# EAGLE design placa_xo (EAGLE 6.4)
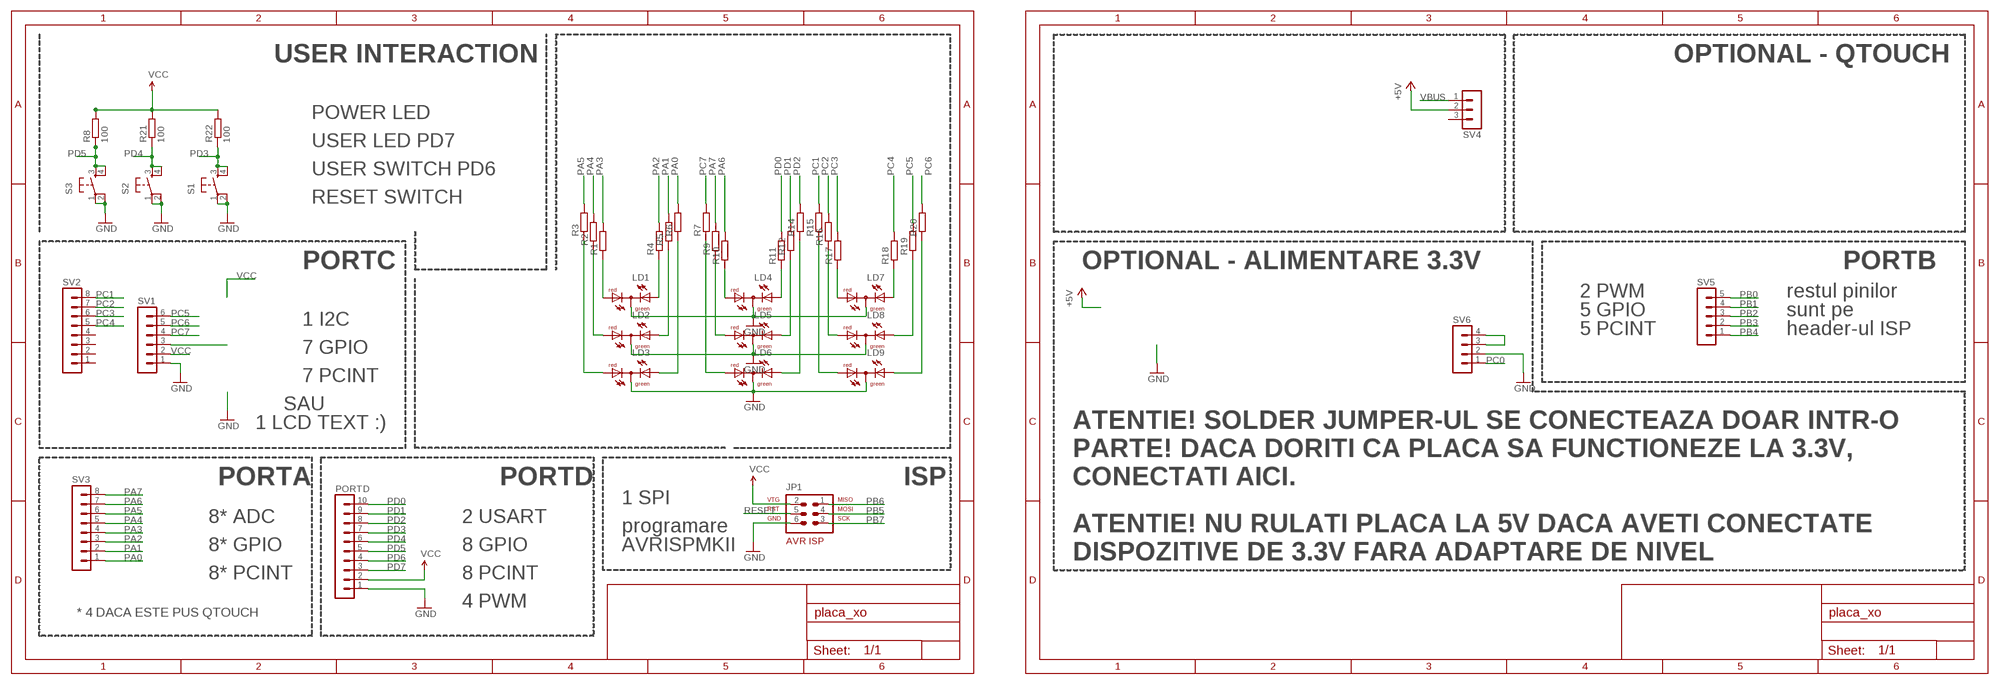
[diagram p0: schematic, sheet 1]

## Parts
JP1  AVR-ISP-6  [AVR-ISP-6]
LD1  DUOLED-RG-C  [DUOLED-C-5MM]
LD2  DUOLED-RG-C  [DUOLED-C-5MM]
LD3  DUOLED-RG-C  [DUOLED-C-5MM]
LD4  DUOLED-RG-C  [DUOLED-C-5MM]
LD5  DUOLED-RG-C  [DUOLED-C-5MM]
LD6  DUOLED-RG-C  [DUOLED-C-5MM]
LD7  DUOLED-RG-C  [DUOLED-C-5MM]
LD8  DUOLED-RG-C  [DUOLED-C-5MM]
LD9  DUOLED-RG-C  [DUOLED-C-5MM]
PORTD  MA10-1W  [MA10-1W]
R1  R-EU_M0805  [M0805]
R2  R-EU_M0805  [M0805]
R3  R-EU_M0805  [M0805]
R4  R-EU_M0805  [M0805]
R5  R-EU_M0805  [M0805]
R6  R-EU_M0805  [M0805]
R7  R-EU_M0805  [M0805]
R8  100  R-EU_0204/7  [0204/7]
R9  R-EU_M0805  [M0805]
R10  R-EU_M0805  [M0805]
R11  R-EU_M0805  [M0805]
R12  R-EU_M0805  [M0805]
R14  R-EU_M0805  [M0805]
R15  R-EU_M0805  [M0805]
R16  R-EU_M0805  [M0805]
R17  R-EU_M0805  [M0805]
R18  R-EU_M0805  [M0805]
R19  R-EU_M0805  [M0805]
R20  R-EU_M0805  [M0805]
R21  100  R-EU_0204/7  [0204/7]
R22  100  R-EU_0204/7  [0204/7]
S1  TAC_SWITCHPTH  [TACTILE-PTH]
S2  TAC_SWITCHPTH  [TACTILE-PTH]
S3  TAC_SWITCHPTH  [TACTILE-PTH]
SV1  MA06-1  [MA06-1]
SV2  MA08-1  [MA08-1]
SV3  MA08-1  [MA08-1]
SV4  MA03-1  [MA03-1]
SV5  MA05-1  [MA05-1]
SV6  MA04-1  [MA04-1]

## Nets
+5V: SV4.2
GND: JP1.6 LD1.C LD2.C LD3.C LD4.C LD5.C LD6.C LD7.C LD8.C LD9.C PORTD.1 S1.1 S1.2 S2.1 S2.2 S3.1 S3.2 SV1.1 SV6.2
N$5: SV6.3 SV6.4
N$7: LD1.AR R1.1
N$8: LD1.AX(AG) R4.1
N$9: LD2.AR R2.1
N$10: LD2.AX(AG) R5.1
N$11: LD3.AR R3.1
N$12: SV1.3
N$13: LD3.AX(AG) R6.1
N$14: LD6.AR R7.1
N$15: LD6.AX(AG) R14.1
N$16: LD5.AX(AG) R12.1
N$18: LD4.AX(AG) R11.1
N$19: LD4.AR R10.1
N$20: LD5.AR R9.1
N$21: LD9.AR R15.1
N$22: LD9.AX(AG) R20.1
N$23: LD8.AX(AG) R19.1
N$24: LD8.AR R16.1
N$25: LD7.AX(AG) R18.1
N$26: LD7.AR R17.1
PA0: R6.2 SV3.1
PA1: R5.2 SV3.2
PA2: R4.2 SV3.3
PA3: R1.2 SV3.4
PA4: R2.2 SV3.5
PA5: R3.2 SV3.6
PA6: R10.2 SV3.7
PA7: R9.2 SV3.8
PB0: SV5.5
PB1: SV5.4
PB2: SV5.3
PB3: SV5.2
PB4: SV5.1
PB5: JP1.4
PB6: JP1.1
PB7: JP1.3
PC0: SV6.1
PC1: R15.2 SV2.8
PC2: R16.2 SV2.7
PC3: R17.2 SV2.6
PC4: R18.2 SV2.5
PC5: R19.2 SV1.6
PC6: R20.2 SV1.5
PC7: R7.2 SV1.4
PD0: PORTD.10 R11.2
PD1: PORTD.9 R12.2
PD2: PORTD.8 R14.2
PD3: PORTD.7 R22.1 S1.3 S1.4
PD4: PORTD.6 R21.1 S2.3 S2.4
PD5: PORTD.5 R8.1 S3.3 S3.4
PD6: PORTD.4
PD7: PORTD.3
RESET: JP1.5
VBUS: SV4.1
VCC: JP1.2 PORTD.2 R8.2 R21.2 R22.2 SV1.2
Unconnected: SV2.1 SV2.2 SV2.3 SV2.4 SV4.3

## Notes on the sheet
- USER INTERACTION | OPTIONAL - QTOUCH
- POWER LED
- USER LED PD7
- USER SWITCH PD6
- RESET SWITCH
- PORTC | OPTIONAL - ALIMENTARE 3.3V | PORTB
- 2 PWM | restul pinilor
- 5 GPIO | sunt pe
- 1 I2C
- 5 PCINT | header-ul ISP
- 7 GPIO
- 7 PCINT
- SAU
- 1 LCD TEXT :) | ATENTIE! SOLDER JUMPER-UL SE CONECTEAZA DOAR INTR-O
- PARTE! DACA DORITI CA PLACA SA FUNCTIONEZE LA 3.3V,
- PORTA | PORTD | ISP | CONECTATI AICI.
- 1 SPI
- 8* ADC | 2 USART
- programare | ATENTIE! NU RULATI PLACA LA 5V DACA AVETI CONECTATE
- 8* GPIO | 8 GPIO | AVRISPMKII
- DISPOZITIVE DE 3.3V FARA ADAPTARE DE NIVEL
- 8* PCINT | 8 PCINT
- 4 PWM
- * 4 DACA ESTE PUS QTOUCH

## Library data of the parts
JP1 = 0andrei_custom:AVR-ISP-6: AVR ISP-6 Serial Programming Header
LD1-LD9 = led:DUOLED-RG-C: DUO LED 2 colors (red/green), 5 mm, round, common Cathode www.ligitek.com or other producers.
PORTD = con-lstb:MA10-1W: PIN HEADER; OC_FARNELL: unknown; OC_NEWARK: unknown
R1-R7 R9-R12 R14-R20 = rcl:R-EU_: RESISTOR, European symbol
R8 R21 R22 = 0andrei_custom:R-EU_: RESISTOR, European symbol
S1-S3 = SparkFun:TAC_SWITCH: Momentary Switch Button commonly used for reset or general input. Spark Fun Electronics SKU : COM-00097
SV1 = con-lstb:MA06-1: PIN HEADER; OC_FARNELL: unknown; OC_NEWARK: unknown
SV2 SV3 = con-lstb:MA08-1: PIN HEADER; OC_FARNELL: unknown; OC_NEWARK: unknown
SV4 = con-lstb:MA03-1: PIN HEADER; OC_FARNELL: unknown; OC_NEWARK: unknown
SV5 = con-lstb:MA05-1: PIN HEADER; OC_FARNELL: unknown; OC_NEWARK: unknown
SV6 = con-lstb:MA04-1: PIN HEADER; OC_FARNELL: unknown; OC_NEWARK: unknown

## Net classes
1 power: width 0.61 mm

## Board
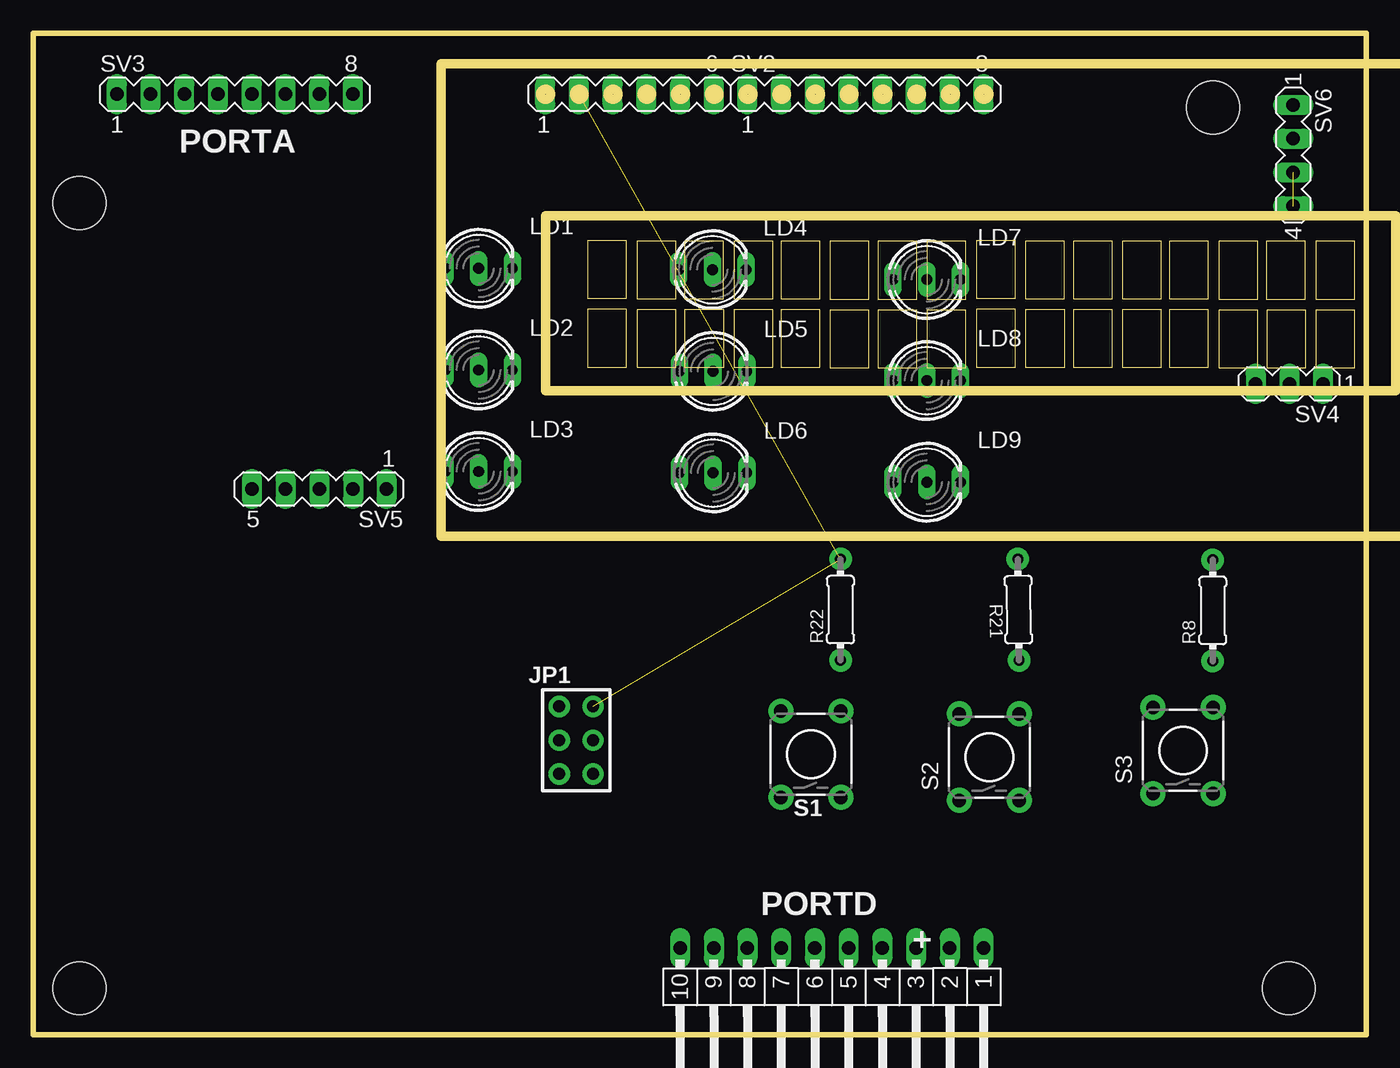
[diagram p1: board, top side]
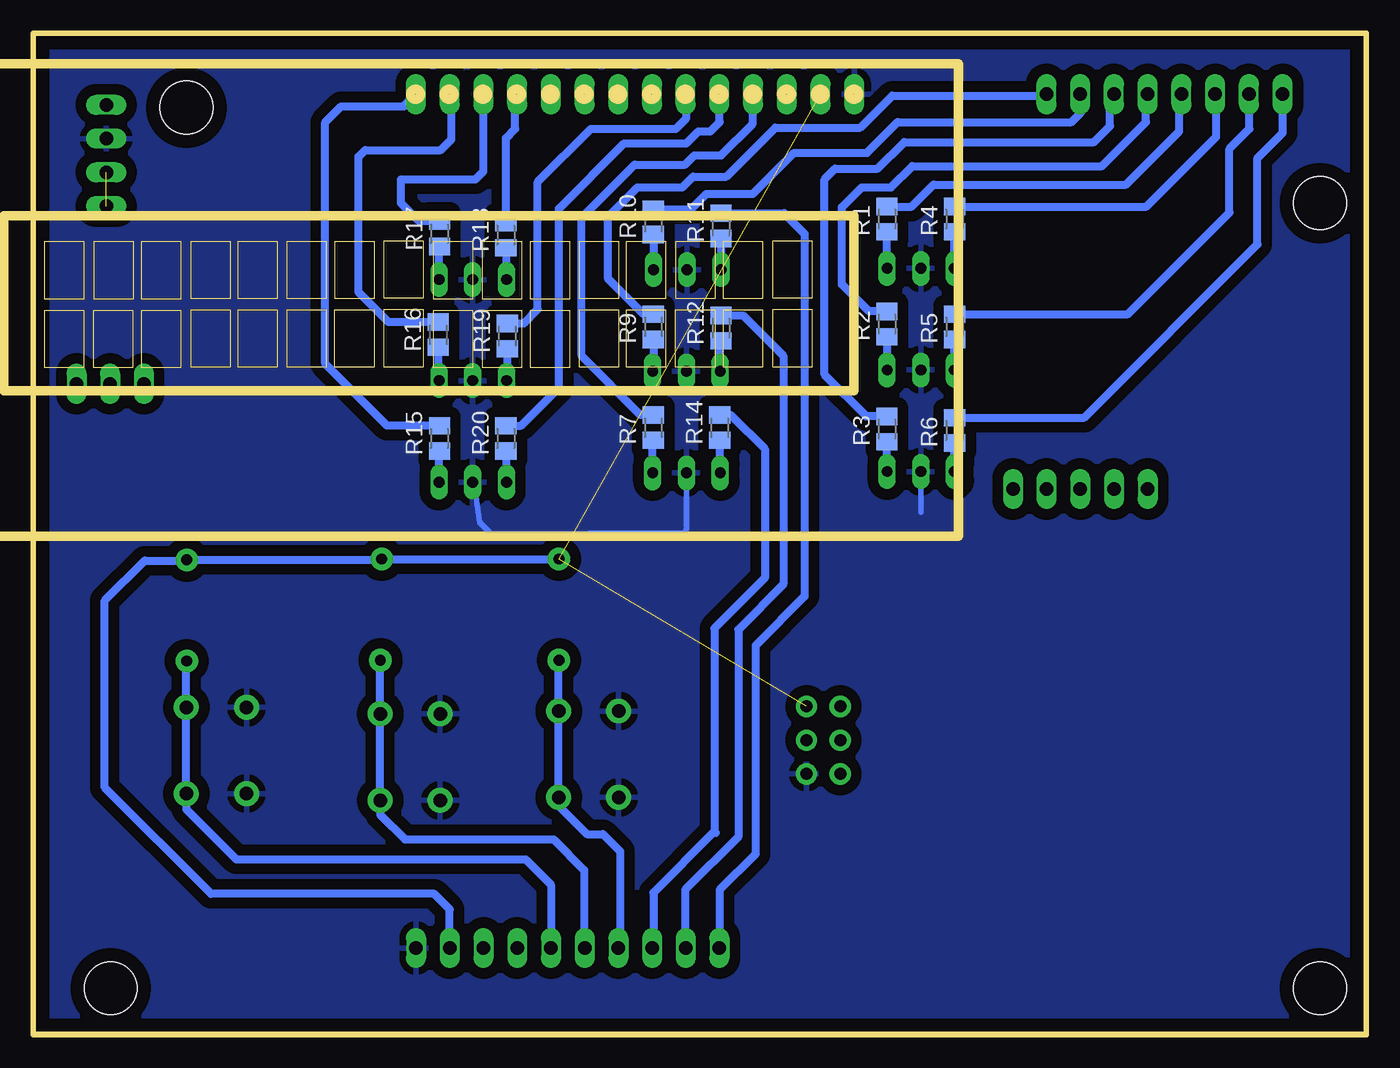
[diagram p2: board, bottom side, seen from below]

Size 100.4 x 75.4 mm. Coordinates in mm from the lower left corner, seen from the top.
Outline: 0.2,0.2 100.2,0.2
Outline: 0,0 100.4,0 100.4,75.4 0,75.4 0,0
Copper layers (1*16): Top 0.035mm / dielectric 1.5mm / Bottom 0.035mm
Design rules "default": minimum track width 10mil, minimum drill 24mil, track to track 0.8mm, track to pad 10mil, pad to pad 10mil, via to via 10mil, smd to smd 0mil, copper to edge 40mil, drill to drill 10mil, minimum pad ring 10mil, minimum via ring 8mil, stop-mask expansion 0mil, vias tented up to drill 0mil, thermal gap 20mil
Holes 4 mm at 88.86,69.8 3.5,3.5 3.5,62.6 94.56,3.5
Milling: area 38.2,70.5 to 39,71.2; area 40.8,70.5 to 41.5,71.2; area 43.3,70.5 to 44,71.2; area 45.9,70.5 to 46.6,71.2; area 48.4,70.5 to 49.1,71.2; area 50.9,70.5 to 51.7,71.2; area 53.5,70.5 to 54.2,71.2; area 56,70.5 to 56.7,71.2; area 58.6,70.5 to 59.3,71.2; area 61.1,70.5 to 61.8,71.2; area 63.6,70.5 to 64.4,71.2; area 66.2,70.5 to 66.9,71.2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; 8 lines

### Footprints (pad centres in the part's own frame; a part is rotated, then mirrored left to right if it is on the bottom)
AVR-ISP-6 = drill 0.9 pad 1.6: 1 -2.54,-1.27; 2 -2.54,1.27; 3 0,-1.27; 4 0,1.27; 5 2.54,-1.27; 6 2.54,1.27
DUOLED-C-5MM = drill 0.813 long: AR 2.54,0; AX -2.54,0; C 0,0
MA10-1W = drill 1.016 long: 1 -11.43,0; 2 -8.89,0; 3 -6.35,0; 4 -3.81,0; 5 -1.27,0; 6 1.27,0; 7 3.81,0; 8 6.35,0; 9 8.89,0; 10 11.43,0
M0805 = smd 1.3 x 1.6: 1 -0.95,0; 2 0.95,0
0204/7 = drill 0.813 pad 1.7: 1 -3.81,0; 2 3.81,0
TACTILE-PTH = drill 1.016 pad 1.88: 1 -3.251,2.261; 2 3.251,2.261; 3 -3.251,-2.261; 4 3.251,-2.261
MA06-1 = drill 1.016 long: 1 -6.35,0; 2 -3.81,0; 3 -1.27,0; 4 1.27,0; 5 3.81,0; 6 6.35,0
MA08-1 = drill 1.016 long: 1 -8.89,0; 2 -6.35,0; 3 -3.81,0; 4 -1.27,0; 5 1.27,0; 6 3.81,0; 7 6.35,0; 8 8.89,0
MA03-1 = drill 1.016 long: 1 -2.54,0; 2 0,0; 3 2.54,0
MA05-1 = drill 1.016 long: 1 -5.08,0; 2 -2.54,0; 3 0,0; 4 2.54,0; 5 5.08,0
MA04-1 = drill 1.016 long: 1 -3.81,0; 2 -1.27,0; 3 1.27,0; 4 3.81,0

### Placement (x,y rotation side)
JP1  40.89,22.18 270 top
LD1  33.55,57.7 0 top
LD2  33.55,50.05 0 top
LD3  33.55,42.4 0 top
LD4  51.15,57.6 0 top
LD5  51.2,49.95 0 top
LD6  51.2,42.3 0 top
LD7  67.3,56.85 0 top
LD8  67.3,49.25 0 top
LD9  67.3,41.6 0 top
PORTD  60.14,6.53 180 top
R1  36.1,61.4 90 bottom
R2  36.1,53.5 90 bottom
R3  36.1,45.6 90 bottom
R4  31,61.4 90 bottom
R5  31,53.3 90 bottom
R6  31,45.5 90 bottom
R7  53.7,45.7 90 bottom
R8  88.83,31.94 90 top
R9  53.7,53.3 90 bottom
R10  53.7,61.2 90 bottom
R11  48.6,60.9 90 bottom
R12  48.6,53.2 90 bottom
R14  48.7,45.7 90 bottom
R15  69.8,44.9 90 bottom
R16  69.9,52.7 90 bottom
R17  69.8,60.3 90 bottom
R18  64.8,60.2 90 bottom
R19  64.7,52.6 90 bottom
R20  64.8,44.9 90 bottom
R21  74.2,32 90.7 top
R22  60.8,32 90 top
S1  58.56,21.12 90 top
S2  72,20.9 90 top
S3  86.6,21.4 90 top
SV1  44.9,70.81 0 top
SV2  62.68,70.81 0 top
SV3  15.19,70.81 0 top
SV4  94.6,49 180 top
SV5  21.54,41.09 180 top
SV6  94.9,66.2 270 top

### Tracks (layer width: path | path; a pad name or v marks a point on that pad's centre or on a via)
GND
  Bottom 0.406: LD3.C 33.55,39.35 | LD9.C 67.2,41.5 66.8,38.6 65.9,37.7 51.3,37.8 51.2,38.1 LD6.C
  pour Bottom (isolate 0.61): 100.4,75.6 100.4,0 0,0 0,75.4
N$5  (1 unrouted)
N$7
  Bottom 0.61: LD1.AR R1.1
N$8
  Bottom 0.61: LD1.AX 31.01,60.64 R4.1
N$9
  Bottom 0.61: R2.1 LD2.AR
N$10
  Bottom 0.61: LD2.AX R5.1
N$11
  Bottom 0.61: LD3.AR R3.1
N$13
  Bottom 0.61: LD3.AX R6.1
N$14
  Bottom 0.61: LD6.AR 53.74,44.71 R7.1
N$15
  Bottom 0.61: LD6.AX 48.66,44.71 R14.1
N$16
  Bottom 0.61: LD5.AX 48.66,52.19 R12.1
N$18
  Bottom 0.61: R11.1 LD4.AX
N$19
  Bottom 0.61: R10.1 LD4.AR
N$20
  Bottom 0.61: R9.1 53.7,49.99 LD5.AR
N$21
  Bottom 0.61: LD9.AR 69.84,43.91 R15.1
N$22
  Bottom 0.61: LD9.AX 64.76,43.91 R20.1
N$23
  Bottom 0.61: R19.1 64.7,49.31 LD8.AX
N$24
  Bottom 0.61: R16.1 69.9,49.31 LD8.AR
N$25
  Bottom 0.61: LD7.AX 64.76,59.21 R18.1
N$26
  Bottom 0.61: LD7.AR 69.84,59.31 R17.1
PA0
  Bottom 0.61: R6.2 21.25,46.45 8.2,59.5 8.2,66 6.3,67.9 SV3.1
PA1
  Bottom 0.61: R5.2 17.95,54.25 10.3,61.9 10.3,66.7 8.8,68.2 8.8,70.78 SV3.2
PA2
  Bottom 0.61: R4.2 16.55,62.35 11.3,67.6 11.3,70.74 SV3.3
PA3
  Bottom 0.61: R1.2 34.25,62.35 32.6,64 18.1,64 14.1,68 14.1,70.63 SV3.4
PA4
  Bottom 0.61: R2.2 37.45,54.45 39.5,56.5 39.5,62.3 38,63.8 35.8,63.8 34.2,65.4 19.9,65.4 16.6,68.7 16.6,70.67 SV3.5
PA5
  Bottom 0.61: R3.2 37.65,46.55 40.8,49.7 40.8,64.4 40,65.2 36.8,65.2 34.8,67.2 20.5,67.2 19.3,68.4 19.3,70.51 SV3.6
PA6
  Bottom 0.61: R10.2 50.85,62.15 49.7,63.3 46.2,63.3 43.1,66.4 37.6,66.4 35.3,68.7 22.2,68.7 21.5,69.4 21.5,70.78 SV3.7
PA7
  Bottom 0.61: R9.2 54.45,54.25 57.1,56.9 57.1,61.6 54.9,63.8 51.5,63.8 50.7,64.6 48.2,64.6 44.5,68.3 38.1,68.3 35.7,70.7 24.19,70.7 SV3.8
PC1
  Bottom 0.61: R15.2 73.75,45.85 78.4,50.5 78.4,68.7 77.2,69.9 72.49,69.9 SV2.8
PC2
  Bottom 0.61: R16.2 73.65,53.65 75.9,55.9 75.9,66.1 75.4,66.6 69.7,66.6 68.9,67.4 68.9,70.68 SV2.7
PC3
  Bottom 0.61: R17.2 71.35,61.25 72.7,62.6 72.7,64.4 67.1,64.4 66.49,65.01 SV2.6
PC4
  Bottom 0.61: R18.2 64.8,67.5 64.1,68.2 64.1,70.67 SV2.5
PC5
  Bottom 0.61: R19.2 63.45,53.55 62.4,54.6 62.4,64.2 58.4,68.2 52,68.2 51.2,69 51.2,70.76 SV1.6
PC6
  Bottom 0.61: R20.2 63.65,45.85 60.8,48.7 60.8,62.2 55.9,67.1 51.2,67.1 50.3,68 49.4,68 48.7,68.7 48.7,70.8 SV1.5
PC7
  Bottom 0.61: R7.2 54.65,46.65 59.1,51.1 59.1,61.5 55.1,65.5 51.3,65.5 50.6,66.2 48.6,66.2 46.2,68.6 46.2,70.79 SV1.4
PD0
  Bottom 0.61: R11.2 43.85,61.85 42.3,60.3 42.3,33 46,29.3 46,13.6 48.7,10.9 PORTD.10
PD1
  Bottom 0.61: R12.2 46.95,54.15 43.9,51.1 43.9,33.9 47.3,30.5 47.3,14.9 51.3,10.9 51.3,6.57 PORTD.9
PD2
  Bottom 0.61: R14.2 47.85,46.65 45.3,44.1 45.3,34.4 49.1,30.6 49.1,15.3 49,15.2 49.2,15.2 53.7,10.7 53.7,6.62 PORTD.8
PD3
  Bottom 0.61: PORTD.7 56.2,6.66 56.2,13.8 57.5,15.1 58.7,15.1 60.82,17.22 S1.3 S1.4 60.82,28.17 R22.1
PD4
  Bottom 0.61: PORTD.6 58.9,6.55 58.9,12.4 61.2,14.7 72.4,14.7 74.26,16.56 S2.3 S2.4 74.26,28.18 R21.1
PD5
  Bottom 0.61: PORTD.5 61.4,11.3 63.3,13.2 85.1,13.2 88.86,16.96 S3.3 S3.4 88.86,28.11 R8.1
VCC  (2 unrouted)
  Bottom 0.61: PORTD.2 69.03,9.43 70.2,10.6 87,10.6 95,18.6 95,32.7 92,35.7 88.89,35.7 R8.2 74.21,35.75 R21.2 R22.2 | R22.2

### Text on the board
tPlace: PORTA | PORTD
tNames: +
_tsilk: Header Compatibil LCD 2x16 | Optional | 1k | alimentare 3.3V | PORTA | 100nF | 10k | PORTC / LCD | BA033 | 100nF | 100u | 100u | 1 | PORTB | MEGA324-P | DCJ0202 | Optional | 7805T | alimentare 12V | Optional | QUARTZ | 100nF | QTouch | 100nF | 15pF | 15pF | 1K | AVR-ISP-6 | BUTON USER | LED | LED | ROTOR | 1K | 3V3 | SPI | 100 | 100 | PORTD | KEY | 100 | 2K2 | 10K | BUTON RESET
